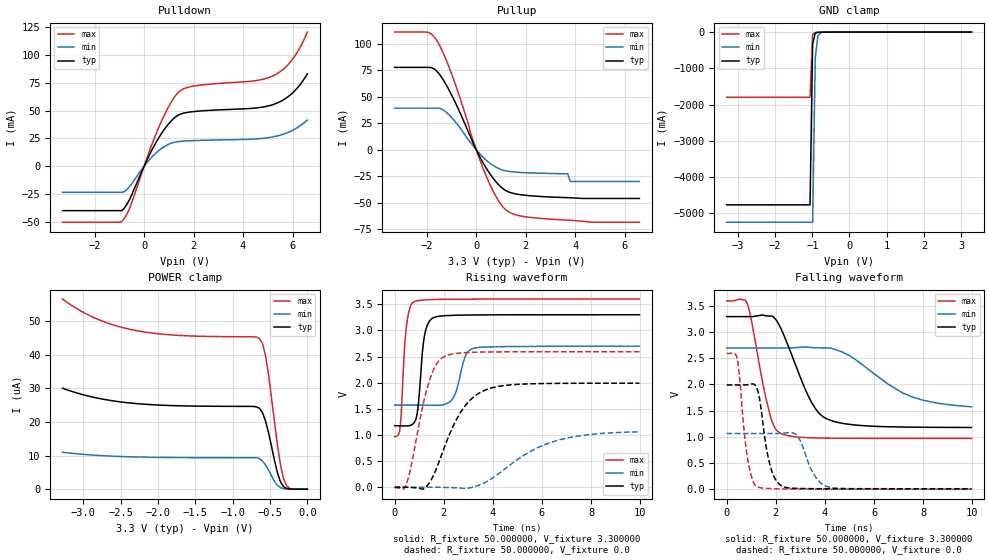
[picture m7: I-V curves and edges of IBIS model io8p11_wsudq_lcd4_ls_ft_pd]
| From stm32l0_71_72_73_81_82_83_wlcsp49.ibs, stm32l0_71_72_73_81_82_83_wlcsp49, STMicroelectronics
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|   Model io8p11_wsudq_lcd4_ls_ft_pd
[Model]  io8p11_wsudq_lcd4_ls_ft_pd
Model_type I/O
Polarity   Non-Inverting
Enable   Active-Low
Vinl =   0.990000V
Vinh =   2.310000V
Vmeas =  1.650000V
Cref =   50.000000pF
Rref =   100.000000M
Vref =   0.0V
C_comp   3.263700pF   3.224800pF   3.309000pF
[Temperature Range]   25.000000   0.125000k   -40.000000
[Pullup Reference]   3.300000V   2.700000V   3.600000V
[Pulldown Reference]   0.0V   0.0V   0.0V
[POWER Clamp Reference]   3.300000V   2.700000V   3.600000V
[GND Clamp Reference]   0.0V   0.0V   0.0V
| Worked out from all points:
|   slope of the pulldown table from 0 to 0.495 V, typ, clamps not added: 22.6 ohm
|   slope of the pullup table from 0 to 0.495 V, typ, clamps not added: 23.9 ohm
|   GND clamp passes 1 mA (typ) near -0.64 V on its own axis
|   rising waveform, R_fixture 50.000000, V_fixture 3.300000: 20-80 % time 240ps typ, 378ps min, 202ps max; typ from 1.18 V to 3.3 V
|   rising waveform, R_fixture 50.000000, V_fixture 0.0: 20-80 % time 1.2ns typ, 2.22ns min, 722ps max; typ from 0 V to 1.99 V
|   falling waveform, R_fixture 50.000000, V_fixture 3.300000: 20-80 % time 1.14ns typ, 2.12ns min, 656ps max; typ from 3.3 V to 1.18 V
|   falling waveform, R_fixture 50.000000, V_fixture 0.0: 20-80 % time 416ps typ, 580ps min, 338ps max; typ from 1.99 V to 0 V
[Pulldown]
|Voltage   I(typ)   I(min)   I(max)
-3.3V     -39.83mA   -23.37mA   -50.2mA
-900mV    -39.83mA   -23.37mA   -49.53mA
-600mV    -30.28mA   -18.59mA   -38.45mA
500mV     22.11mA    12.28mA    30.1mA
1V        38.33mA    19.81mA    53.88mA
1.4V      46.1mA     22.18mA    66.72mA
2V        49.07mA    23.02mA    71.93mA
4.4V      52.05mA    24.38mA    76.53mA
5.2V      55.25mA    26.3mA     81.02mA
5.6V      59.18mA    28.57mA    86.57mA
6V        65.79mA    32.24mA    95.97mA
6.6V      82.83mA    41.41mA    120.4mA
[Pullup]
|Voltage   I(typ)   I(min)   I(max)
-3.3V     77.63mA    39.16mA    110.9mA
-2V       77.63mA    39.16mA    110.9mA
-1.6V     74.23mA    39.16mA    103.3mA
-1.3V     64.67mA    36.99mA    89.45mA
-900mV    47.14mA    27.82mA    65.37mA
300mV     -13.29mA   -7.65mA    -18.99mA
800mV     -30.32mA   -16.54mA   -44.19mA
1.2V      -38.62mA   -20mA      -56.79mA
1.9V      -42.8mA    -21.61mA   -62.92mA
3.7V      -45.29mA   -22.8mA    -66.51mA
3.8V      -45.39mA   -30mA      -66.64mA
6.6V      -46mA      -30mA      -68.41mA
[GND_clamp]
|Voltage   I(typ)   I(min)   I(max)
-3.3V     -4.767A    -5.246A    -1.798A
-1.06V    -4.767A    -5.246A    -1.798A
-990mV    -327.3mA   -5.246A    -68.39mA
-920mV    -29.24mA   -722.7mA   -11.25mA
-850mV    -6.784mA   -104.5mA   -6.73mA
-780mV    -3.572mA   -17.39mA   -4.335mA
-500mV    -70.03uA   -187.2uA   -42.37uA
3.28V     73.94uA    88.61uA    51.47uA
[POWER_clamp]
|Voltage   I(typ)   I(min)   I(max)
-3.28V    30.09uA    10.99uA    56.63uA
-2.84V    27.27uA    10.11uA    50.92uA
-2.32V    25.55uA    9.609uA    47.36uA
-640mV    24.06uA    9.1uA      44.84uA
-600mV    22.76uA    8.366uA    43.37uA
-560mV    20.32uA    7.212uA    39.74uA
-520mV    16.86uA    5.676uA    34.15uA
-400mV    4.842uA    1.146uA    13.11uA
-360mV    2.185uA    478.4nA    7.29uA
-320mV    773nA      181.6nA    3.214uA
-240mV    60.58nA    0A         296.5nA
0V        0A         0A         0A
[Ramp]
| variable   typ   min   max
dV/dt_r  1.19316/1.19367n   0.60876/2.08480n   1.55490/0.71965n
dV/dt_f  1.27164/1.13248n   0.59250/1.87506n   1.57816/0.65481n
R_load = 50.000000
[Rising Waveform]
R_fixture= 50.000000
V_fixture= 3.300000
V_fixture_min= 2.700000
V_fixture_max= 3.600000
|time   V(typ)   V(min)   V(max)
0s        1.176V     1.571V     966.1mV
220.2ps   1.175V     1.571V     1.129V
460.5ps   1.172V     1.571V     2.985V
780.8ps   1.227V     1.571V     3.544V
940.9ps   1.483V     1.571V     3.567V
1.221ns   2.908V     1.57V      3.583V
1.582ns   3.242V     1.566V     3.591V
2.342ns   3.287V     1.679V     3.597V
3.183ns   3.295V     2.652V     3.598V
9.97ns    3.299V     2.698V     3.599V
[Rising Waveform]
R_fixture= 50.000000
V_fixture= 0.0
V_fixture_min= 0.0
V_fixture_max= 0.0
|time   V(typ)   V(min)   V(max)
0s        163.8uV    9.237uV    -5.567mV
360.4ps   31.99uV    -4.13uV    -37.18mV
480.5ps   -997uV     -7.784uV   64.93mV
1.361ns   49.44mV    175.8uV    1.953V
1.662ns   311.1mV    -250.7uV   2.319V
2.002ns   731.6mV    -2.636mV   2.494V
2.843ns   1.539V     -23.3mV    2.573V
3.804ns   1.879V     120.5mV    2.587V
6.386ns   1.985V     860.5mV    2.591V
9.97ns    1.99V      1.06V      2.592V
[Falling Waveform]
R_fixture= 50.000000
V_fixture= 3.300000
V_fixture_min= 2.700000
V_fixture_max= 3.600000
|time   V(typ)   V(min)   V(max)
0s        3.299V     2.698V     3.599V
860.9ps   3.298V     2.698V     3.517V
1.702ns   3.31V      2.698V     1.535V
1.922ns   3.285V     2.698V     1.206V
2.162ns   3.113V     2.698V     1.074V
3.323ns   1.78V      2.714V     980mV
3.984ns   1.365V     2.7V       972.2mV
5.005ns   1.235V     2.55V      968.2mV
7.568ns   1.182V     1.758V     966.4mV
9.97ns    1.176V     1.571V     966.1mV
[Falling Waveform]
R_fixture= 50.000000
V_fixture= 0.0
V_fixture_min= 0.0
V_fixture_max= 0.0
|time   V(typ)   V(min)   V(max)
0s        1.99V      1.06V      2.592V
420.4ps   1.99V      1.06V      2.507V
840.8ps   1.994V     1.06V      607.1mV
1.241ns   1.913V     1.06V      38.87mV
1.762ns   461.6mV    1.06V      6.939mV
2.302ns   41.91mV    1.067V     -599.4uV
2.883ns   9.077mV    1.008V     -3.299mV
3.504ns   4.1mV      316.6mV    -4.244mV
4.064ns   2.537mV    47.89mV    -4.707mV
9.97ns    163.8uV    9.237uV    -5.567mV
